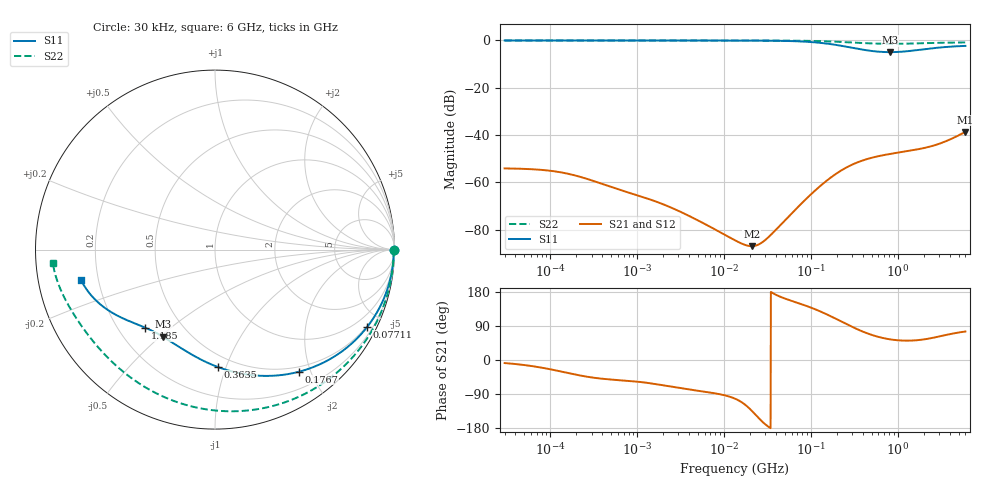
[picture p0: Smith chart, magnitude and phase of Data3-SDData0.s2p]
!EMIF06-MSD04F3
!Simulation
!24/03/11  09:25
!Start Freq. :30.000kHz; Stop Freq. : 6.000GHz
!Number of points : 1592; Sweep : LOGARITHMIC
!D1-A4 (Data3-SDData0)
!Freq ReS11 ImS11 ReS21 ImS21 ReS12 ImS12 ReS22 ImS22
# Hz  S  RI  R  50
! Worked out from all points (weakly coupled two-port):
!   1592 points, 30 kHz to 6 GHz, reference 50 ohm
!   highest |S21| = -38.67 dB at 6 GHz (marker M1); lowest = -87.0 dB at 20.91 MHz (marker M2)
!   lowest |S11| = -5.0 dB at 813.7 MHz (marker M3), VSWR 3.60, Z = 17.9 - j25.6 ohm
!   |S11| at or under -10 dB: nowhere
!   |S22| runs from -1.4 to 0.0 dB; largest |S21 - S12| = 1.3e-14
!   S11 on the Smith chart (normalised r, x): 30 kHz: open; 77.11 MHz: 0.46, -4.12; 176.7 MHz: 0.43, -1.83; 363.5 MHz: 0.41, -0.94; 1.185 GHz: 0.31, -0.41; 6 GHz: 0.13, -0.11
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30000  0.998 -0.000465  0.00195 -0.000276  0.00195 -0.000276  0.998 -0.000464
97078.1  0.9976 -0.00132  0.00162 -0.000713  0.00162 -0.000713  0.9976 -0.00132
150356.2  0.9973 -0.00179  0.00131 -0.000846  0.00131 -0.000846  0.9973 -0.00179
231093.6  0.997 -0.0023  0.000956 -0.00085  0.000956 -0.00085  0.997 -0.0023
1766531  0.9961 -0.0114  0.00016 -0.000339  0.00016 -0.000339  0.9961 -0.0114
3340319  0.9958 -0.0212  5.8e-05 -0.00022  5.8e-05 -0.00022  0.9958 -0.0212
7830472  0.9943 -0.0492  3.89e-06 -0.000102  3.89e-06 -0.000102  0.9947 -0.0492
1.350376e7  0.9909 -0.0845  -1.26e-05 -5.77e-05  -1.26e-05 -5.77e-05  0.992 -0.0846
2.091484e7  0.9838 -0.1302  -3.1e-05 -3.21e-05  -3.1e-05 -3.21e-05  0.9865 -0.1306
3.985241e7  0.9528 -0.2423  -9.92e-05 1.41e-05  -9.92e-05 1.41e-05  0.9619 -0.2453
7.711187e7  0.8475 -0.4314  -0.000295 0.000186  -0.000295 0.000186  0.8748 -0.4509
1.032257e8  0.7517 -0.5319  -0.000429 0.000398  -0.000429 0.000398  0.79 -0.5728
1.350376e8  0.6266 -0.618  -0.000532 0.000732  -0.000532 0.000732  0.6706 -0.6925
1.766531e8  0.4687 -0.6802  -0.00053 0.00122  -0.00053 0.00122  0.5037 -0.8022
2.553414e8  0.2273 -0.7015  -0.000183 0.00204  -0.000183 0.00204  0.207 -0.8935
3.634583e8  0.0164 -0.6543  0.000544 0.00269  0.000544 0.00269  -0.1011 -0.8804
5.375942e8  -0.1588 -0.5674  0.00149 0.00307  0.00149 0.00307  -0.3903 -0.7658
7.890804e8  -0.2801 -0.491  0.00226 0.00323  0.00226 0.00323  -0.5854 -0.6139
8.136818e8  -0.2885 -0.4859  0.00231 0.00324  0.00231 0.00324  -0.5975 -0.6018
1.18519e9  -0.3876 -0.4354  0.00279 0.00347  0.00279 0.00347  -0.7156 -0.464
2.757113e9  -0.6148 -0.324  0.00307 0.00539  0.00307 0.00539  -0.8574 -0.2291
6e9  -0.7474 -0.1678  0.00298 0.0113  0.00298 0.0113  -0.9036 -0.0764
